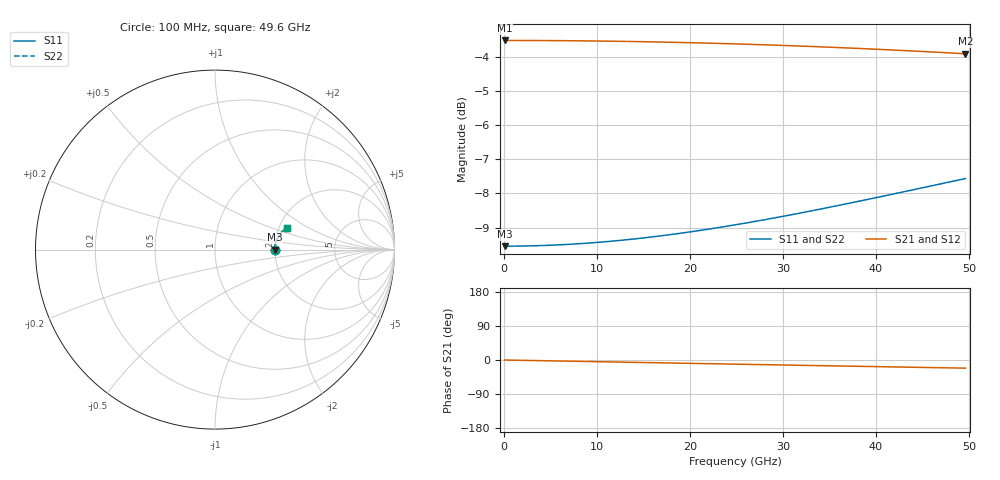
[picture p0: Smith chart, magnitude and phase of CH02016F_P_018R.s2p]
# GHz S RI R 18
! S-Parameters data
! Freq  reS11  imS11  reS21  imS21  reS12  imS12  reS22  imS22
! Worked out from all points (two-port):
!   100 points, 100 MHz to 49.6 GHz, reference 18 ohm
!   highest |S21| = -3.52 dB at 100 MHz (marker M1); lowest = -3.9 dB at 49.6 GHz (marker M2)
!   |S21| within 3 dB of the highest: start of sweep to end of sweep
!   lowest |S11| = -9.5 dB at 100 MHz (marker M3), VSWR 2.00, Z = 36 + j0.0234 ohm
!   |S11| at or under -10 dB: nowhere
!   |S22| runs from -9.5 to -7.6 dB; largest |S21 - S12| = 0
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0.1  0.3333 0.000289  0.6667 -0.000516  0.6667 -0.000516  0.3333 0.000289
2.1  0.3335 0.00608  0.6665 -0.0108  0.6665 -0.0108  0.3335 0.00608
4.1  0.3338 0.0119  0.6661 -0.0211  0.6661 -0.0211  0.3338 0.0119
6.1  0.3344 0.0176  0.6655 -0.0314  0.6655 -0.0314  0.3344 0.0176
8.6  0.3355 0.0248  0.6643 -0.0442  0.6643 -0.0442  0.3355 0.0248
10.6  0.3367 0.0305  0.663 -0.0544  0.663 -0.0544  0.3367 0.0305
12.6  0.3381 0.0361  0.6615 -0.0646  0.6615 -0.0646  0.3381 0.0361
14.6  0.3397 0.0417  0.6598 -0.0747  0.6598 -0.0747  0.3397 0.0417
16.6  0.3415 0.0472  0.6578 -0.0847  0.6578 -0.0847  0.3415 0.0472
18.6  0.3436 0.0526  0.6555 -0.0947  0.6555 -0.0947  0.3436 0.0526
20.6  0.3459 0.0579  0.653 -0.1045  0.653 -0.1045  0.3459 0.0579
22.6  0.3484 0.0632  0.6503 -0.1143  0.6503 -0.1143  0.3484 0.0632
25.1  0.3518 0.0696  0.6466 -0.1264  0.6466 -0.1264  0.3518 0.0696
27.1  0.3548 0.0747  0.6434 -0.1359  0.6434 -0.1359  0.3548 0.0747
29.1  0.3579 0.0796  0.6399 -0.1453  0.6399 -0.1453  0.3579 0.0796
31.1  0.3613 0.0843  0.6362 -0.1546  0.6362 -0.1546  0.3613 0.0843
33.1  0.3649 0.089  0.6323 -0.1638  0.6323 -0.1638  0.3649 0.089
37.1  0.3725 0.0979  0.624 -0.1816  0.624 -0.1816  0.3725 0.0979
39.1  0.3766 0.1021  0.6195 -0.1904  0.6195 -0.1904  0.3766 0.1021
41.6  0.382 0.1072  0.6136 -0.201  0.6136 -0.201  0.382 0.1072
45.6  0.391 0.1147  0.6037 -0.2176  0.6037 -0.2176  0.391 0.1147
49.6  0.4006 0.1216  0.5931 -0.2335  0.5931 -0.2335  0.4006 0.1216
